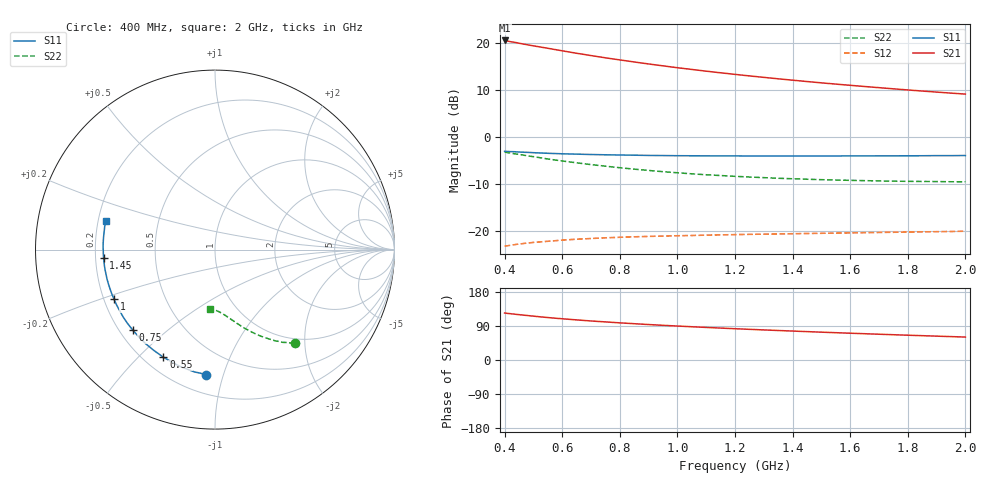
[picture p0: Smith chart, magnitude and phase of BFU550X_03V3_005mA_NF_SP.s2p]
! Filename:  P:\Prog\Test\Noise\ATS_data\Testdata_Net\BFU550X no attenuator noise\BFU550X_APG2013_44_C05_03p3V_005mA_NF_CM01_D.sf
! Date/Time: Fri 26/Jul/2013 14:37:11
! BFU550X_APG2013_44_C05_03p3V_1to10mA_NF_CM01_Bias4_R.sf
! Noise Parameter Data File
! BFU550X_APG2013_44_C05_03p3V_1to10mA_NF_CM01
! Date/time: Wed Jul 24 15:50:55 2013
! VAR V_out= 3.300000
! VAR I_out= 5.005000
! VAR V_in= 0.816100
! VAR I_in= 0.055905
! Device data file deembeded for feedlines and parallel
! Original file: \BFU550X no attenuator noise\BFU550X_APG2013_44_C05_03p3V_005mA_NF_CM01_R.sf
! Feed-files: PR005V01_100713_Feed1.s2p, PR005V01_100713_Feed2.s2p
! Parallel-file: PR005V01_100713_Par.s2p
# MHz S MA R 50
!  Freq-MHz  S11-mag  S11-arg  S21-mag  S21-arg  S12-mag  S12-arg  S22-mag  S22-arg
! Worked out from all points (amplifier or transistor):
!   37 points, 400 MHz to 2 GHz, reference 50 ohm
!   highest |S21| = 20.5 dB at 400 MHz (marker M1)
!   |S21| within 3 dB of that: start of sweep to 678.1 MHz
!   unconditionally stable (mu >= 1): nowhere
!   at 500 MHz: K = 0.27, MSG = 20.9 dB, |S12| = -22.5 dB
!   at 1.1 GHz: K = 0.56, MSG = 17.4 dB, |S12| = -21.0 dB
!   at 2 GHz: K = 0.90, MSG = 14.6 dB, |S12| = -20.1 dB
!   lowest NFmin = 0.64 dB at 433 MHz
!   S11 on the Smith chart (normalised r, x): 400 MHz: 0.32, -0.87; 550 MHz: 0.28, -0.59; 750 MHz: 0.25, -0.38; 1 GHz: 0.24, -0.22; 1.45 GHz: 0.23, -0.03; 2 GHz: 0.23, +0.12
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400  0.6986 -94.3  10.55 123.9  0.06831 45.5  0.6851 -49.6
420  0.6925 -97.4  10.25 122.2  0.06977 44.4  0.6674 -51.1
440  0.6888 -100.6  10.01 120.5  0.0713 43.2  0.6536 -52.4
460  0.6834 -103.3  9.727 118.8  0.07258 42.1  0.6399 -53.9
500  0.6748 -109.0  9.247 115.7  0.07491 40.1  0.6123 -56.3
550  0.6649 -115.7  8.71 112.0  0.07699 38.0  0.5782 -59.2
600  0.6568 -121.3  8.189 108.8  0.07917 36.2  0.551 -61.6
650  0.6513 -126.5  7.71 105.8  0.08104 34.7  0.5267 -63.8
700  0.6453 -131.4  7.288 103.0  0.08242 33.4  0.5039 -65.9
750  0.641 -135.7  6.896 100.5  0.08383 32.2  0.4849 -67.7
800  0.6377 -139.9  6.551 98.0  0.08492 31.2  0.4666 -69.5
850  0.6347 -143.8  6.228 95.8  0.08593 30.4  0.4509 -71.0
900  0.6309 -147.4  5.933 93.6  0.08677 29.7  0.4367 -72.5
950  0.629 -150.7  5.662 91.5  0.08749 29.1  0.4237 -74.0
1000  0.6267 -153.8  5.412 89.6  0.08821 28.6  0.4125 -75.2
1100  0.6245 -159.6  4.972 86.0  0.08946 27.8  0.393 -77.7
1200  0.6236 -164.8  4.597 82.5  0.09069 27.2  0.3781 -80.0
1300  0.6226 -169.4  4.271 79.4  0.0917 26.9  0.3661 -82.0
1450  0.6227 -175.9  3.858 74.9  0.09318 26.7  0.3522 -85.0
1500  0.6226 -177.9  3.734 73.5  0.09363 26.7  0.3483 -85.9
1750  0.6248 173.0  3.225 66.7  0.09597 27.0  0.336 -90.3
2000  0.6296 165.2  2.835 60.5  0.09858 27.9  0.3308 -94.4
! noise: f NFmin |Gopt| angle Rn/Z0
400  0.6774  0.1593  38.4  0.1131
460  0.654  0.1207  62.64  0.0897
600  0.7284  0.158  65.81  0.104
800  0.7274  0.1766  90.8  0.0907
1000  0.7776  0.2188  108.3  0.0819
1200  0.7996  0.2669  125.4  0.0714
1400  0.852  0.2912  137.6  0.0664
1600  0.8651  0.3347  149.7  0.0556
1800  0.8932  0.3563  160.2  0.0513
2000  0.9331  0.431  171.1  0.0391
